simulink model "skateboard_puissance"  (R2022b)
settings: Solver=FixedStepAuto  StartTime=0.0  StopTime=1  FixedStep=0.001  RelTol=1e-3
libraries: fl_lib x10, nesl_utility x6, batteryecm_lib x1, ee_lib x1, sdl_lib x1

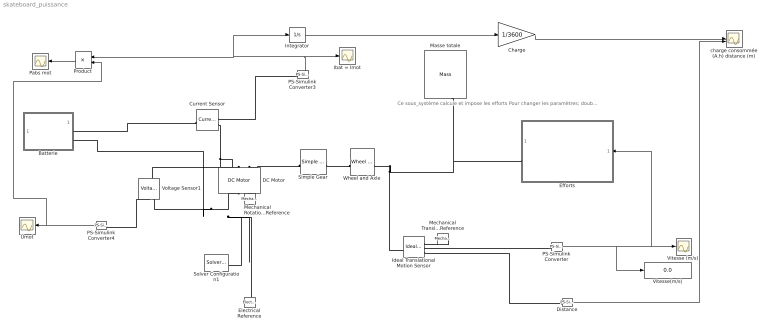
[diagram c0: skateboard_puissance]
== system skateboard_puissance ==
  note: Ce sous_système calcule et impose les efforts Pour changer les paramètres; double cliquez (Dans la zone blanche ci-dessus)
  Batterie : Subsystem  mask{Tension=1, cap=1}
      mask prompts: Tension "Tension (V)"; cap "Capacité (A.h)"
  Charge : Gain  Gain=1/3600
  Current Sensor : fl_lib/Electrical/Electrical Sensors/Current Sensor
  DC Motor : ee_lib/Electromechanical/Brushed Motors/DC Motor  field_option=ee.enum.field_option.pm  Rf=100 Ohm  Lf=1 H  Laf=0.15 H  If0=0 A  parameterization=ee.enum.dcparam_option.circuit_param  Ra=0.2 Ohm  La=2e-4 H  emf_or_torque=1  Kv=0.082 V/(rad/s)  Ki=6.876e-4 N*m/A  T_stall=0.24e-3 N*m  w_max=4600 rpm  w_rated=4100 rpm  P_rated=600 W  V_rated=36 V  lam_param=2  i_noload=2 A  V_i_noload=36 V  J=10 g*cm^2  lam=0 N*m/(rad/s)  speed0=0 rad/s  enable_fault_armature=simscape.enum.onoff.off  rev_faulted=1 / 3  G_faulted_armature=1e-5 S  fault_trigger_armature=ee.enum.faults.faultTrigger.temporal  t_fault_armature=1 s  max_permissible_current_armature=inf A  t_fail_on_current_armature=1 s  enable_fault_field=simscape.enum.onoff.off  G_faulted_field=1e-5 S  fault_trigger_field=ee.enum.faults.faultTrigger.temporal  t_fault_field=1 s  max_permissible_current_field=inf A  t_fail_on_current_field=1 s  fault_action=simscape.enum.assert.action.none  alpha=3.93e-3 1/K  Tmeas=25 degC  thermal_mass=100 J/K  initial_temperature=25 degC
  Distance : nesl_utility/PS-Simulink Converter  PhysicalDomain=network_engine_domain  SubClassName=ps_output  LeftPortType=input  RightPortType=output  PseudoPeriodic=off  Frequencies=[]  VectorFormat=1-D array  Unit=1  AffineConversion=off
  Efforts : Subsystem  mask{masse=60, angle=0, Cx=0.3, S=1, rho=1.2, Ravancement=0}
      mask prompts: masse "masse totale (kg)"; angle "angle pente (degré)"; Cx "Cx (Sans unité)"; S "Surface frontale S (m^2)"; rho "Masse volumique de l'air (kg/m^3)"; Ravancement "Résistance à l'avancement (N)"
  Electrical Reference : fl_lib/Electrical/Electrical Elements/Electrical Reference
  Ibat = Imot : Scope
  Ideal Translational Motion Sensor : fl_lib/Mechanical/Mechanical Sensors/Ideal Translational Motion Sensor  reference=foundation.enum.MeasurementReference.difference  acceleration_port=false  velocity_port=true  position_port=true  offset=0 m
  Integrator : Integrator
  Masse totale : fl_lib/Mechanical/Translational Elements/Mass  mass=80 kg  num_ports=foundation.enum.numPorts2.one  v_specify=on  v_priority=None  v=0 m/s  v_nominal_specify=off  v_nominal_unit=m/s  v_nominal_value=1  f_specify=off  f_priority=None  f=0 N  f_nominal_specify=off  f_nominal_unit=N  f_nominal_value=1
  Mechanical Rotational Reference : fl_lib/Mechanical/Rotational Elements/Mechanical Rotational Reference
  Mechanical Translational Reference : fl_lib/Mechanical/Translational Elements/Mechanical Translational Reference
  PS-Simulink Converter : nesl_utility/PS-Simulink Converter  PhysicalDomain=network_engine_domain  SubClassName=ps_output  LeftPortType=input  RightPortType=output  PseudoPeriodic=off  Frequencies=[]  VectorFormat=1-D array  Unit=1  AffineConversion=off
  PS-Simulink Converter3 : nesl_utility/PS-Simulink Converter  PhysicalDomain=network_engine_domain  SubClassName=ps_output  LeftPortType=input  RightPortType=output  PseudoPeriodic=off  Frequencies=[]  VectorFormat=1-D array  Unit=1  AffineConversion=off
  PS-Simulink Converter4 : nesl_utility/PS-Simulink Converter  PhysicalDomain=network_engine_domain  SubClassName=ps_output  LeftPortType=input  RightPortType=output  PseudoPeriodic=off  Frequencies=[]  VectorFormat=1-D array  Unit=1  AffineConversion=off
  Pabs mot : Scope
  Product : Product
  Simple Gear : sdl_lib/Gears/Simple Gear  ratio=43/16  rotation_direction=3-2*(1)  friction_model=2  T_noload=0.1 N*m  T_nom=5 N*m  efficiency_nom=0.8  efficiency=0.9  temperature_TLU=[280, 300, 320] K  load_TLU=[1, 5, 10] N*m  efficiency_TLU=[.95, .9, .85]  efficiency_TLU2=[.85, .8, .75; .95, .9, .85; .85, .8, .7]  w_thr=0.01 rad/s  pwr_thr=0.001 W  backlash_model=sdl.enum.backlashModel.Off  backlash_distance=1e-3 mm  x0=0 mm  r_base=0.1 m  hardstop_model=simscape.enum.hardstop.smooth  transition=1e-4 mm  backlash_stiffness=1e7 N/m  backlash_damping=1e6 N*s/m  e=0  v_tol=0.001 m/s  mu_visc=[0, 0] N*m/(rad/s)  enable_faults=0  efficiency_fault=0.05  external_fault=simscape.enum.onoff.off  temporal_fault=0  fault_time=5 s  fault_angles=pi / 12 rad  report_fault=(1)-1  thermal_mass=50 J/K  temperature_specify=off  temperature_priority=High  temperature=300 K  temperature_nominal_specify=off  temperature_nominal_unit=K  temperature_nominal_value=1  x_backlash_specify=off  x_backlash_priority=None  x_backlash=0 mm  x_backlash_nominal_specify=off  x_backlash_nominal_unit=mm  x_backlash_nominal_value=1  f_hardstop_specify=off  f_hardstop_priority=None  f_hardstop=0 N  f_hardstop_nominal_specify=off  f_hardstop_nominal_unit=N  f_hardstop_nominal_value=1  v_backlash_specify=off  v_backlash_priority=None  v_backlash=0 m/s  v_backlash_nominal_specify=off  v_backlash_nominal_unit=m/s  v_backlash_nominal_value=1
  Solver Configuration1 : nesl_utility/Solver Configuration  PhysicalDomain=network_engine_domain  SubClassName=solver  LeftPortType=input  RightPortType=generic  Tones=[]  Harmonics=[]  SimulateNoise=off  Profile=off  UseLocalSampling=off  EnableSwitchedLinearOptims=on  FrequencyDomain=off  UseCCode=off  RelTol=0.001  AbsTol=1e-06  MinStep=1e-09  ToWorkspace=off  RevertToSquareIcSolve=off  NumHomotopyIterations=100  PhasorMode=off  PhasorModeNumHarmonics=1  ConsistencySolver=NEWTON_FTOL  IndexReductionMethod=DerivativeReplacement  DoDC=off  ResidualTolerance=1e-09  ConsistencyTolSource=GLOBAL  ConsistencyAbsTol=0.001  ConsistencyRelTol=0.001  ConsistencyTolFactor=0.001  UseLocalSolver=off  LocalSolverChoice=NE_BACKWARD_EULER_ADVANCER  ResolveIndetEquations=on  FunctionEvalNumThread=1  LocalSolverSampleTime=0.001  DoFixedCost=off  MaxNonlinIter=3  MaxModeIter=2  ComputeImpulses=off  ImpulseIterations=2  LinearAlgebra=auto  LinearAlgebraNumThread=0  EquationFormulation=NE_TIME_EF  DelaysMemoryBudget=1024  AutomaticFiltering=on  FilteringTimeConstant=0.001  PartitionStorageMethod=AS_NEEDED  PartitionMemoryBudget=1024  PartitionMethod=FAST
  Umot : Scope
  "Vitesse (m/s) " : Scope
  Vitesse(m/s) : Display
  Voltage Sensor1 : fl_lib/Electrical/Electrical Sensors/Voltage Sensor
  Wheel and Axle : fl_lib/Mechanical/Mechanisms/Wheel and Axle  R=0.054 m  or=1  t_specify=off  t_priority=None  t=0 N*m  t_nominal_specify=off  t_nominal_unit=N*m  t_nominal_value=1  f_specify=off  f_priority=None  f=0 N  f_nominal_specify=off  f_nominal_unit=N  f_nominal_value=1
  charge consommée (A.h) distance (m) : Scope  NumInputPorts=2
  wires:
  PS-Simulink Converter3/1 -> Integrator/1, Product/1, Ibat = Imot/1
  PS-Simulink Converter/1 -> Vitesse(m/s)/1, "Vitesse (m/s) "/1, Efforts/1(vitesse)
  PS-Simulink Converter4/1 -> Product/2, Umot/1
  Integrator/1 -> Charge/1
  Charge/1 -> charge consommée (A.h) distance (m)/1
  Distance/1 -> charge consommée (A.h) distance (m)/2
  Product/1 -> Pabs mot/1
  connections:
  PS-Simulink Converter3/LConn1 -- Current Sensor/RConn1
  Current Sensor/RConn2 -- Voltage Sensor1/LConn1 -- DC Motor/LConn1
  Simple Gear/LConn1 -- DC Motor/LConn2
  Wheel and Axle/LConn1 -- Simple Gear/RConn1
  Efforts/RConn1 -- Ideal Translational Motion Sensor/LConn1 -- Wheel and Axle/RConn1 -- Masse totale/LConn1
  PS-Simulink Converter/LConn1 -- Ideal Translational Motion Sensor/RConn2
  Mechanical Translational Reference/LConn1 -- Ideal Translational Motion Sensor/RConn1
  Ideal Translational Motion Sensor/RConn3 -- Distance/LConn1
  PS-Simulink Converter4/LConn1 -- Voltage Sensor1/RConn1
  Voltage Sensor1/RConn2 -- Batterie/RConn2 -- Solver Configuration1/RConn1 -- Electrical Reference/LConn1 -- DC Motor/RConn1
  Mechanical Rotational Reference/LConn1 -- DC Motor/RConn2
  Batterie/RConn1 -- Current Sensor/LConn1

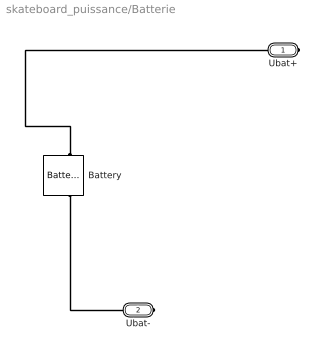
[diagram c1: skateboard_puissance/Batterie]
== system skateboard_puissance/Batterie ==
  Battery : batteryecm_lib/Battery  Vnom=Tension V  prm_dir=simscape.enum.battery.prm_dir.disabled  R1_dis=2 Ohm  R1_ch=2 Ohm  R1=0.03 Ohm  prm_AH=2  AH=cap hr*A  V1=33 V  AH1=3.9 hr*A  prm_R2=1  R2=2000 Ohm  prm_dyn=1  Rp1=0.005 Ohm  tau1=30 s  Rp2=0.005 Ohm  tau2=30 s  Rp3=0.005 Ohm  tau3=30 s  Rp4=0.005 Ohm  tau4=30 s  Rp5=0.005 Ohm  tau5=30 s  prm_fade=1  N_fade=100  AH_fade=45 hr*A  R1_fade=2.02 Ohm  R1_ch_fade=2.02 Ohm  V1_fade=10.35 V  prm_age=simscape.enum.battery.prm_age.disabled  prm_age_OCV=simscape.enum.battery.prm_age_OCV.OCV  OCV_age=0.9  SOC_age=60  delta_time_age_vec=[0] d  temperature_age_vec=[273] K  OCV_scaling_age=2.2134e6  OCV_offset_age=1.632e6  temp_exp_age=0.515833569 V  t_exp_age=0.75  i_specify=off  i_priority=None  i=0 A  i_nominal_specify=off  i_nominal_unit=A  i_nominal_value=1  v_specify=off  v_priority=None  v=0 V  v_nominal_specify=off  v_nominal_unit=V  v_nominal_value=1  charge_specify=on  charge_priority=High  charge=cap hr*A  charge_nominal_specify=off  charge_nominal_unit=A*hr  charge_nominal_value=1  num_cycles_specify=on  num_cycles_priority=None  num_cycles=0  num_cycles_nominal_specify=off  num_cycles_nominal_unit=1  num_cycles_nominal_value=1  Tmeas=298.15 K  Tmeas_age=298.15 K  Vnom_T2=12 V  R1_T2=2.2 Ohm  R1_T2_dis=2.2 Ohm  R1_T2_ch=2.2 Ohm  V1_T2=11.4 V  R2_T2=2200 Ohm  Rp1_T2=0.005 Ohm  tau1_T2=30 s  Rp2_T2=0.005 Ohm  tau2_T2=30 s  Rp3_T2=0.005 Ohm  tau3_T2=30 s  Rp4_T2=0.005 Ohm  tau4_T2=30 s  Rp5_T2=0.005 Ohm  tau5_T2=30 s  Tmeas2=273.15 K  thermal_mass=30000 J/K  temperature_specify=off  temperature_priority=High  temperature=298.15 K  temperature_nominal_specify=off  temperature_nominal_unit=K  temperature_nominal_value=1
  Ubat+ : PMIOPort  Side=Right
  Ubat- : PMIOPort  Port=2  Side=Right
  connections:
  Battery/LConn1 -- Ubat+/RConn1
  Battery/RConn1 -- Ubat-/RConn1

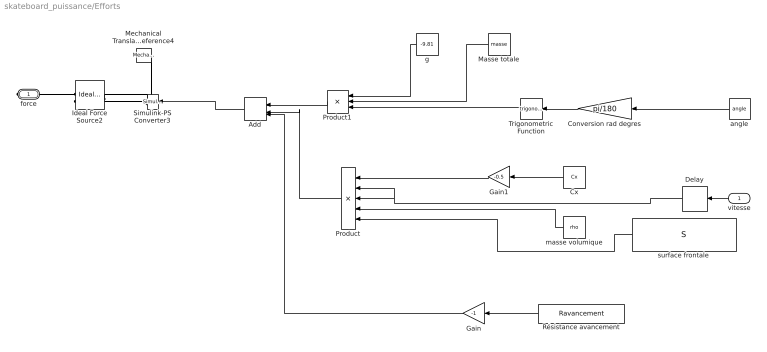
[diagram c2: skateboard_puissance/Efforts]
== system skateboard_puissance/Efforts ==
  vitesse : Inport
  Add : Sum  Inputs=3
  Conversion rad degres : Gain  Gain=pi/180
  Cx : Constant  Value=Cx
  Delay : Delay  DelayLength=1
  Gain : Gain  Gain=-1
  Gain1 : Gain  Gain=-0.5
  Ideal Force Source2 : fl_lib/Mechanical/Mechanical Sources/Ideal Force Source
  Masse totale : Constant  Value=masse
  Mechanical Translational Reference4 : fl_lib/Mechanical/Translational Elements/Mechanical Translational Reference
  Product : Product  Inputs=5
  Product1 : Product  Inputs=3
  Résistance avancement : Constant  Value=Ravancement
  Simulink-PS Converter3 : nesl_utility/Simulink-PS Converter  PhysicalDomain=network_engine_domain  SubClassName=ps_input  LeftPortType=input  RightPortType=output  PseudoPeriodic=off  Frequencies=[]  NoiseDistribution=none  NoiseParameters=[]  Unit=1  AffineConversion=off  FilteringAndDerivatives=filter  SimscapeFilterOrder=1  InputFilterTimeConstant=0.001  UdotUserProvided=1
  Trigonometric Function : Trigonometry
  angle : Constant  Value=angle
  g : Constant  Value=-9.81
  masse volumique : Constant  Value=rho
  surface frontale : Constant  Value=S
  force : PMIOPort  Side=Right
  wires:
  Gain1/1 -> Product/1
  Delay/1 -> Product/2, Product/3
  Gain/1 -> Add/3
  Résistance avancement/1 -> Gain/1
  Product/1 -> Add/2
  Add/1 -> Simulink-PS Converter3/1
  Product1/1 -> Add/1
  vitesse/1 -> Delay/1
  Cx/1 -> Gain1/1
  surface frontale/1 -> Product/5
  masse volumique/1 -> Product/4
  Conversion rad degres/1 -> Trigonometric Function/1
  Trigonometric Function/1 -> Product1/3
  g/1 -> Product1/1
  angle/1 -> Conversion rad degres/1
  Masse totale/1 -> Product1/2
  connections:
  Simulink-PS Converter3/RConn1 -- Ideal Force Source2/RConn1
  Mechanical Translational Reference4/LConn1 -- Ideal Force Source2/RConn2
  Ideal Force Source2/LConn1 -- force/RConn1
